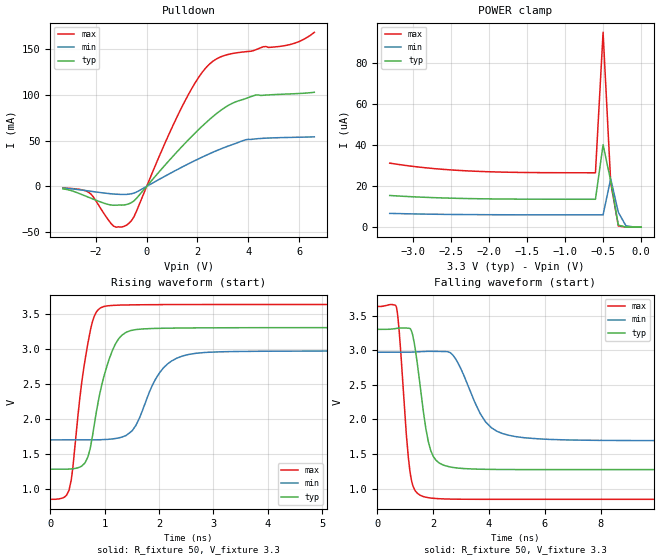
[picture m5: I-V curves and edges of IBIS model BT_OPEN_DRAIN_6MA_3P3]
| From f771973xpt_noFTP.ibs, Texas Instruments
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|BT_WEAK_PU_ON_3P3
|   Model Cell BT_OPEN_DRAIN_6MA_3P3
|BT_OPEN_DRAIN_6MA_3P3
[Model]   BT_OPEN_DRAIN_6MA_3P3
Model_type   I/O_open_drain
Polarity   Inverting
Enable   Active-Low
Vinl =  0.8
Vinh =  2
Cref =  15.0000pF
Rref =  100.0000M
Vref =  0V
Vmeas =  1.65
C_comp   3.98845p   2.03906p   4.55356p
[Model Spec]
Vinl   0.8   0.8   0.8
Vinh   2   2   2
[Temperature Range]   25   155   -40
[Voltage Range]   3.3   2.97   3.63
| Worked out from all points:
|   slope of the pulldown table from 0 to 0.495 V, typ, clamps not added: 30.9 ohm
|   rising waveform, R_fixture 50, V_fixture 3.3: 20-80 % time 345ps typ, 467ps min, 263ps max; typ from 1.28 V to 3.3 V
|   falling waveform, R_fixture 50, V_fixture 3.3: 20-80 % time 422ps typ, 899ps min, 301ps max; typ from 3.3 V to 1.28 V
| Nom Voltages:
|   BIASFET=3.3, VDD=1.2, VDDS=3.3, VSS=0
| Min Voltages:
|   BIASFET=2.97, VDD=1.08, VDDS=2.97, VSS=0
| Max Voltages:
|   BIASFET=3.63, VDD=1.32, VDDS=3.63, VSS=0
[POWER_clamp]
|   voltage   I(typ)   I(min)   I(max)
-3.3V     15.41uA    6.707uA    31.17uA
-2.8V     14.47uA    6.332uA    28.78uA
-2.2V     13.87uA    6.102uA    27.25uA
-1.6V     13.64uA    6.016uA    26.64uA
-600mV    13.58uA    5.99uA     26.46uA
-500mV    40.13uA    5.991uA    94.82uA
-400mV    22.54uA    23.52uA    21.76uA
-300mV    969.1nA    7.215uA    616.4nA
-200mV    29.93nA    661.1nA    11.88nA
0V        1.388nA    48.32nA    1.243nA
[Pulldown]
|   voltage   I(typ)   I(min)   I(max)
-3.3V     -2.737mA   -1.873mA   -1.718mA
-2.3V     -11.76mA   -4.954mA   -6.193mA
-1.3V     -20.63mA   -8.362mA   -43.49mA
-800mV    -19.88mA   -8.768mA   -42.58mA
-500mV    -15.9mA    -7.318mA   -33.21mA
1.4V      43.88mA    21.19mA    87.52mA
1.9V      58.17mA    28.19mA    112.9mA
2.4V      71.33mA    34.76mA    131.7mA
3V        84.76mA    41.87mA    142.6mA
4.3V      99.91mA    51.98mA    149.5mA
5.8V      101.3mA    53.65mA    156.4mA
6.6V      102.9mA    54.17mA    168.5mA
[Ramp]
| variable   typ   min   max
dV/dt_f  1.2265162/0.42596978n 0.77333606/0.9075597n  1.6862307/0.30383977n
dV/dt_r  1.1726677/0.72864722n 0.73282855/1.5166001n  1.5979937/0.48603734n
R_load = 50
[Rising Waveform]
R_fixture = 50
V_fixture = 3.3
V_fixture_min = 2.97
V_fixture_max = 3.63
|   time   V(typ)   V(min)   V(max)
0s        1.279V     1.698V     849.6mV
345.1ps   1.281V     1.698V     978.7mV
635.1ps   1.364V     1.698V     2.818V
807ps     1.906V     1.698V     3.458V
1.046ns   2.76V      1.705V     3.61V
1.258ns   3.141V     1.726V     3.621V
1.47ns    3.256V     1.806V     3.624V
2.083ns   3.291V     2.727V     3.629V
2.855ns   3.297V     2.946V     3.63V
20.09ns   3.3V       2.97V      3.63V
[Falling Waveform]
R_fixture = 50
V_fixture = 3.3
V_fixture_min = 2.97
V_fixture_max = 3.63
|   time   V(typ)   V(min)   V(max)
0s        3.3V       2.97V      3.63V
685.1ps   3.313V     2.97V      3.627V
1.166ns   3.314V     2.971V     1.274V
1.615ns   2.234V     2.98V      893.3mV
1.83ns    1.68V      2.984V     872mV
2.187ns   1.383V     2.982V     857.8mV
2.8ns     1.303V     2.878V     850.5mV
3.881ns   1.281V     1.963V     848.6mV
4.946ns   1.278V     1.754V     848.5mV
20.09ns   1.279V     1.697V     849mV
